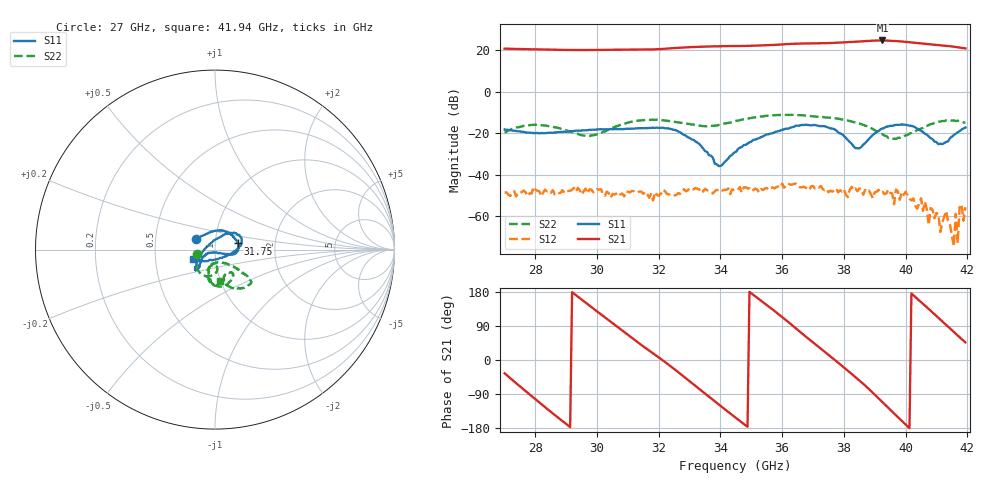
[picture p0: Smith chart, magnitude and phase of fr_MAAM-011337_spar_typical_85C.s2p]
! Created Thu Jan 25 15:58:15 2024
# hz S db R 50
! 2 Port Network Data from SP1.SP block
! freq  dbS11  angS11  dbS21  angS21  dbS12  angS12  dbS22  angS22
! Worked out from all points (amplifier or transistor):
!   240 points, 27 GHz to 41.94 GHz, reference 50 ohm
!   highest |S21| = 24.7 dB at 39.25 GHz (marker M1)
!   |S21| within 3 dB of that: 33.44 GHz to 41.56 GHz (8.119 GHz wide, 21.7 % of centre)
!   unconditionally stable (mu >= 1): start of sweep to end of sweep
!   at 29.5 GHz: K = 14.82, MAG = 20.1 dB, |S12| = -49.7 dB
!   at 34.5 GHz: K = 9.15, MAG = 22.1 dB, |S12| = -47.5 dB
!   at 41.94 GHz: K = 26.51, MAG = 21.0 dB, |S12| = -55.8 dB
!   S11 on the Smith chart (normalised r, x): 27 GHz: 0.80, +0.10; 31.75 GHz: 1.29, +0.09; 41.94 GHz: 0.77, -0.08
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2.70046e10  -18.29 149.7  20.72 -35.2  -48.65 -77.5  -19.85 -165.1
2.806689e10  -19.96 118.5  20.35 -107.9  -47.82 -103.7  -16.08 -111.8
2.881674e10  -19.53 87.0  20.13 -157.2  -48.89 -132.3  -17.84 -87.0
2.95041e10  -18.74 65.5  20.05 159.2  -49.66 -163.5  -21.03 -87.0
3.062888e10  -18.08 37.1  20.19 89.2  -49.20 166.3  -16.75 -107.4
3.175365e10  -17.54 14.9  20.30 21.1  -49.44 134.8  -13.57 -79.9
3.20036e10  -17.54 8.7  20.47 6.6  -50.26 127.0  -13.74 -72.6
3.269096e10  -19.67 -15.3  21.17 -35.7  -49.39 140.3  -14.98 -55.2
3.337832e10  -26.33 -28.5  21.63 -80.6  -46.58 100.6  -16.53 -58.7
3.45031e10  -29.09 -149.9  21.96 -153.1  -47.53 71.6  -14.12 -73.3
3.525295e10  -22.45 -149.2  22.20 160.4  -48.61 57.3  -12.24 -60.5
3.606529e10  -18.19 -135.0  22.81 109.2  -46.40 37.7  -11.29 -46.2
3.70026e10  -16.11 -135.8  23.25 46.0  -45.53 -4.4  -11.95 -40.1
3.762748e10  -17.87 -144.5  23.47 5.3  -48.24 -18.3  -12.69 -39.3
3.812738e10  -23.43 -171.7  23.81 -28.1  -50.86 -27.6  -13.97 -41.0
3.881474e10  -22.86 69.5  24.47 -76.8  -47.75 -53.7  -17.18 -42.3
3.925215e10  -17.84 46.8  24.66 -111.3  -48.35 -70.8  -20.53 -55.4
3.95021e10  -16.51 37.0  24.53 -131.3  -48.86 -88.8  -22.46 -69.9
4.012698e10  -16.38 14.3  23.81 -179.8  -51.74 -103.4  -20.28 -104.9
4.087682e10  -22.96 -32.4  22.72 125.3  -57.15 -137.1  -15.48 -98.9
4.137672e10  -24.05 -115.0  21.98 88.1  -62.34 -76.2  -14.03 -89.8
4.193911e10  -17.33 -156.9  20.83 46.6  -55.76 -20.3  -15.00 -80.8
